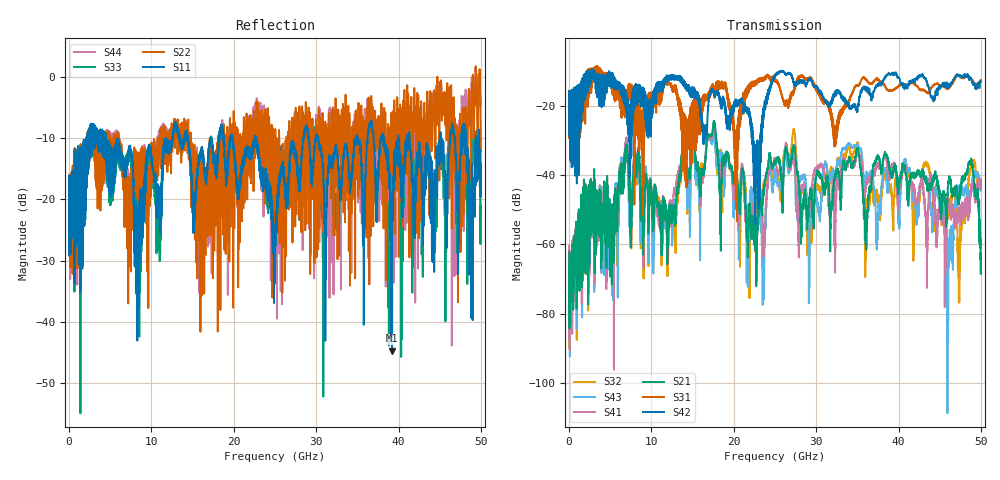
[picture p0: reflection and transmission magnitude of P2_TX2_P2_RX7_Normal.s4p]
!Keysight Technologies,N5225B,MY57041031,A.13.20.10
!Date: Friday, May 31, 2019 11:37:36
!Correction: S11(Full 4 Port(1,2,3,4))
!S12(Full 4 Port(1,2,3,4))
!S13(Full 4 Port(1,2,3,4))
!S14(Full 4 Port(1,2,3,4))
!S21(Full 4 Port(1,2,3,4))
!S22(Full 4 Port(1,2,3,4))
!S23(Full 4 Port(1,2,3,4))
!S24(Full 4 Port(1,2,3,4))
!S31(Full 4 Port(1,2,3,4))
!S32(Full 4 Port(1,2,3,4))
!S33(Full 4 Port(1,2,3,4))
!S34(Full 4 Port(1,2,3,4))
!S41(Full 4 Port(1,2,3,4))
!S42(Full 4 Port(1,2,3,4))
!S43(Full 4 Port(1,2,3,4))
!S44(Full 4 Port(1,2,3,4))
!S4P File: Measurements: <S11,S12,S13,S14>,
!<S21,S22,S23,S24>,
!<S31,S32,S33,S34>,
!<S41,S42,S43,S44>:
# Hz S  dB  R 50.0
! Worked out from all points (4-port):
!   5000 points, 10 MHz to 50 GHz, reference 50 ohm
!   strongest paths, dB at 10 MHz, 12.51 GHz, 25.01 GHz, 37.51 GHz, 50 GHz:
!     S42: -19.5, -12.1, -11.7, -13.7, -13.0
!     S31: -19.4, -14.8, -13.0, -12.4, -12.6
!     S21: -62.1, -52.2, -36.2, -34.6, -62.5
!     S41: -60.4, -52.8, -35.6, -36.5, -43.7
!     S43: -65.4, -60.4, -38.9, -51.2, -43.8
!     S32: -64.8, -57.6, -39.8, -48.3, -41.5
!   lowest |S11| = -44.8 dB at 39.22 GHz (marker M1), VSWR 1.01, Z = 49.9 + j0.575 ohm
!   |S11| at or under -10 dB: 4.481 GHz to 11.72 GHz (7.238 GHz wide, 89.4 % of centre); 22.73 GHz to 28.43 GHz (5.703 GHz wide, 22.3 % of centre); 30.26 GHz to 34.82 GHz (4.561 GHz wide, 14 % of centre)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
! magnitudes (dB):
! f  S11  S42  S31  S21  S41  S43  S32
! 10 MHz  -19.1  -19.5  -19.4  -62.1  -60.4  -65.4  -64.8
! 6.88 GHz  -14.3  -19.7  -18.9  -32.2  -30.4  -30.5  -31.9
! 23.55 GHz  -17.3  -22.3  -11.9  -47.2  -58.9  -67.6  -45.0
! 39.22 GHz  -44.8  -10.6  -15.7  -40.8  -37.3  -38.8  -47.9
! 47.38 GHz  -15.6  -11.4  -11.3  -47.3  -49.3  -43.3  -76.7
! 48.76 GHz  -21.9  -11.8  -12.2  -36.7  -44.9  -46.1  -38.2
! 50 GHz  -14.1  -13.0  -12.6  -62.5  -43.7  -43.8  -41.5
